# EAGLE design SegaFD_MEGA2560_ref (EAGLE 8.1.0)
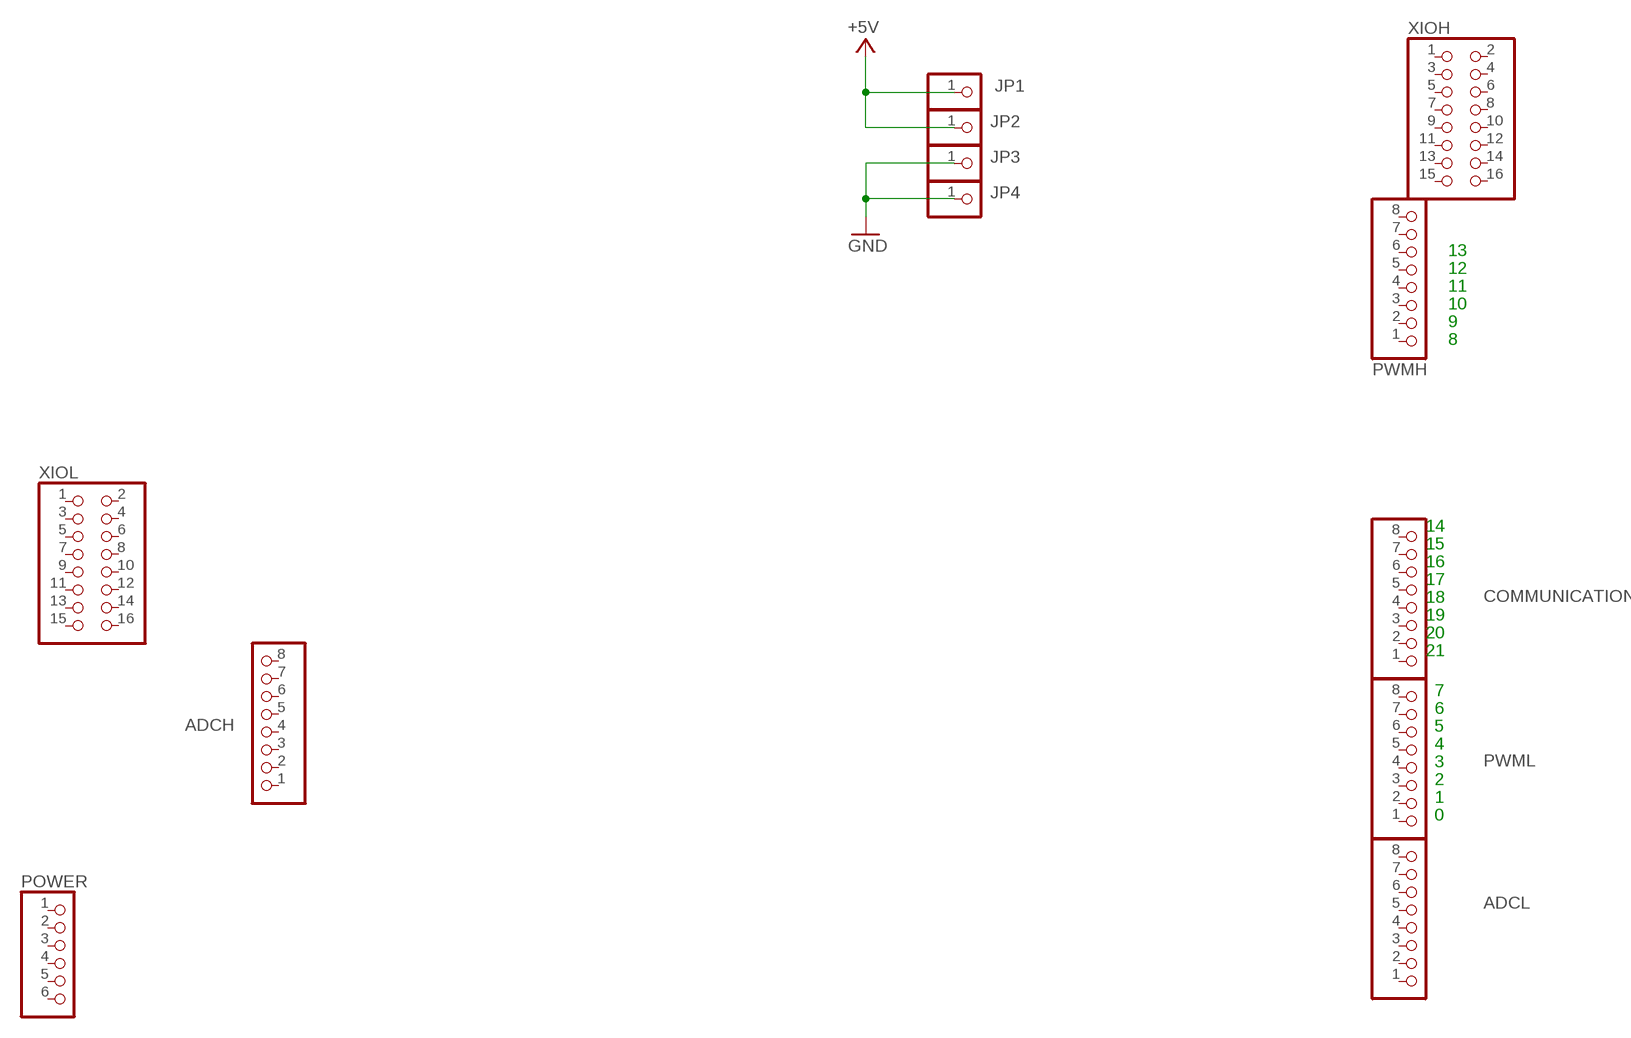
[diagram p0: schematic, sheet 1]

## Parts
ADCH  PINHD-1X8  [1X08]
ADCL  PINHD-1X8  [1X08]
COMMUNICATION  PINHD-1X8  [1X08]
JP1  PINHD-1X1  [1X01]
JP2  PINHD-1X1  [1X01]
JP3  PINHD-1X1  [1X01]
JP4  PINHD-1X1  [1X01]
POWER  PINHD-1X6  [1X06]
PWMH  PINHD-1X8  [1X08]
PWML  PINHD-1X8  [1X08]
XIOH  PINHD-2X8  [2X08]
XIOL  PINHD-2X8  [2X08]

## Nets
+5V: JP1.1 JP2.1
GND: JP3.1 JP4.1
Unconnected: ADCH.1 ADCH.2 ADCH.3 ADCH.4 ADCH.5 ADCH.6 ADCH.7 ADCH.8 ADCL.1 ADCL.2 ADCL.3 ADCL.4 ADCL.5 ADCL.6 ADCL.7 ADCL.8 COMMUNICATION.1 COMMUNICATION.2 COMMUNICATION.3 COMMUNICATION.4 COMMUNICATION.5 COMMUNICATION.6 COMMUNICATION.7 COMMUNICATION.8 POWER.1 POWER.2 POWER.3 POWER.4 POWER.5 POWER.6 PWMH.1 PWMH.2 PWMH.3 PWMH.4 PWMH.5 PWMH.6 PWMH.7 PWMH.8 PWML.1 PWML.2 PWML.3 PWML.4 PWML.5 PWML.6 PWML.7 PWML.8 XIOH.1 XIOH.2 XIOH.3 XIOH.4 XIOH.5 XIOH.6 XIOH.7 XIOH.8 XIOH.9 XIOH.10 XIOH.11 XIOH.12 XIOH.13 XIOH.14 XIOH.15 XIOH.16 XIOL.1 XIOL.2 XIOL.3 XIOL.4 XIOL.5 XIOL.6 XIOL.7 XIOL.8 XIOL.9 XIOL.10 XIOL.11 XIOL.12 XIOL.13 XIOL.14 XIOL.15 XIOL.16

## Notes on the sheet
- 13
- 12
- 11
- 10
- 9
- 8
- 14
- 15
- 16
- 17
- 18
- 19
- 20
- 21
- 7
- 6
- 5
- 4
- 3
- 2
- 1
- 0

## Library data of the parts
ADCH ADCL COMMUNICATION PWMH PWML = pinhead:PINHD-1X8: PIN HEADER
JP1-JP4 = pinhead:PINHD-1X1: PIN HEADER
POWER = pinhead:PINHD-1X6: PIN HEADER
XIOH XIOL = pinhead:PINHD-2X8: PIN HEADER

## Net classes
0 default: width 0.15 mm, drill 0.3 mm, clearance 0.15 mm

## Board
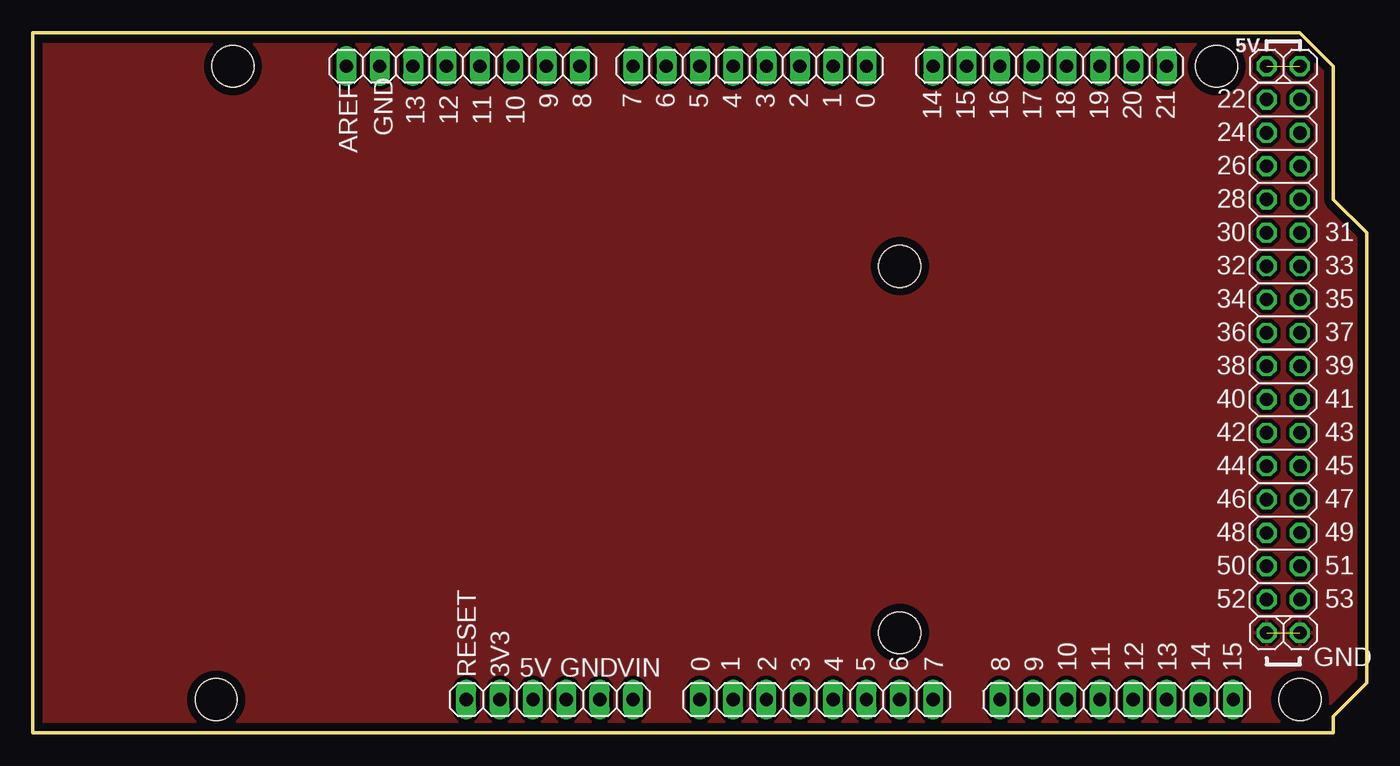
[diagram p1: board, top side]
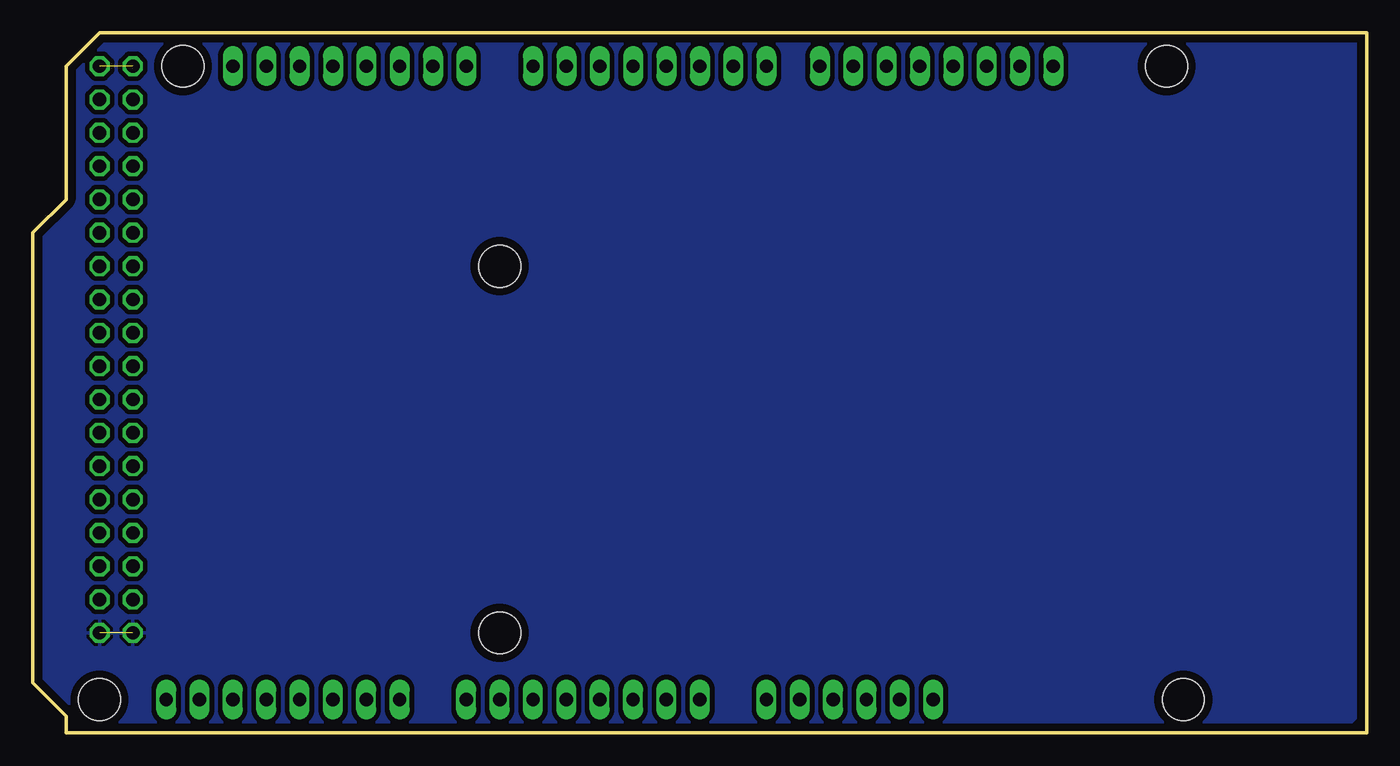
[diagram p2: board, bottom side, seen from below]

Size 101.6 x 53.34 mm. Coordinates in mm from the lower left corner, seen from the top.
Outline: 0,53.34 96.52,53.34 99.06,50.8 99.06,40.64 101.6,38.1 101.6,3.81 99.06,1.27 99.06,0 0,0 0,53.34
Copper layers (1*16): Top 0.035mm / dielectric 1.5mm / Bottom 0.035mm
Design rules "default *": minimum track width 0.15mm, minimum drill 0.3mm, track to track 0.15mm, track to pad 0.15mm, pad to pad 0.15mm, via to via 0.15mm, smd to smd 0.15mm, copper to edge 0.6mm, drill to drill 0.3mm, minimum pad ring 10mil, minimum via ring 10mil, stop-mask expansion 2mil, vias tented up to drill 1mil, thermal gap 10mil
Holes 3.2 mm at 96.52,2.54 15.24,50.8 90.17,50.8 13.97,2.54 66.04,35.56 66.04,7.62

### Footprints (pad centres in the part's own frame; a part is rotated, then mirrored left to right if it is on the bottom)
1X08 = drill 1.016 long: 1 -8.89,0; 2 -6.35,0; 3 -3.81,0; 4 -1.27,0; 5 1.27,0; 6 3.81,0; 7 6.35,0; 8 8.89,0
1X01 = drill 1.016 octagon: 1 0,0
1X06 = drill 1.016 long: 1 -6.35,0; 2 -3.81,0; 3 -1.27,0; 4 1.27,0; 5 3.81,0; 6 6.35,0
2X08 = drill 1.016 octagon: 1 -8.89,-1.27; 2 -8.89,1.27; 3 -6.35,-1.27; 4 -6.35,1.27; 5 -3.81,-1.27; 6 -3.81,1.27; 7 -1.27,-1.27; 8 -1.27,1.27; 9 1.27,-1.27; 10 1.27,1.27; 11 3.81,-1.27; 12 3.81,1.27; 13 6.35,-1.27; 14 6.35,1.27; 15 8.89,-1.27; 16 8.89,1.27

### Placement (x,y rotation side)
ADCH  82.55,2.54 0 top
ADCL  59.69,2.54 0 top
COMMUNICATION  77.47,50.8 180 top
JP1  93.98,50.8 0 top
JP2  96.52,50.8 0 top
JP3  93.98,7.62 0 top
JP4  96.52,7.62 0 top
POWER  39.37,2.54 0 top
PWMH  32.77,50.8 180 top
PWML  54.61,50.8 180 top
XIOH  95.25,39.37 90 top
XIOL  95.25,19.05 90 top

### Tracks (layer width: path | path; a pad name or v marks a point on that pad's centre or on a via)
+5V  (1 unrouted)
GND  (1 unrouted)
  pour Top (isolate 0.305, rank 2): 0.64,52.7 101.6,52.7 101.6,0.64 0.64,0.64
  pour Bottom (isolate 0.356, rank 2): 0.64,52.7 101.6,52.7 102.23,52.07 102.23,0.64 1.27,0.64 0.64,1.27

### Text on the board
tPlace: 9 | 8 | 7 | 6 | 5 | 4 | 3 | 2 | 1 | 0 | 22 | 14 | 15 | 16 | 17 | 18 | 19 | 20 | 21 | 13 | 12 | 11 | 10 | 24 | 26 | 28 | 30 | 31 | 32 | 33 | 34 | 35 | 36 | 37 | 38 | 39 | 40 | 41 | 42 | 43 | 44 | 45 | 46 | 47 | 48 | 49 | 50 | 51 | 52 | 53 | 0 | 1 | 2 | 3 | 4 | 5 | 6 | 7 | 8 | 9 | 10 | 11 | 12 | 13 | 14 | 15
tNames: 5V | GND | AREF | GND | RESET | 3V3 | 5V | GND | VIN
ReferenceLC: L | TX | RX | PC1 | PC2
